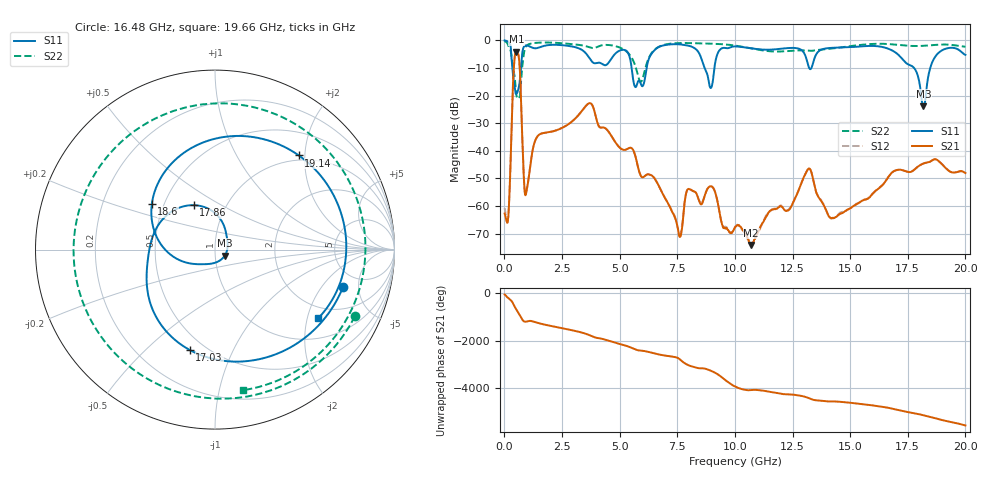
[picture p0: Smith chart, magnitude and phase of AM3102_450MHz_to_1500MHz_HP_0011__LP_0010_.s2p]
!Agilent Technologies,E8364B,MY43040894,A.07.50.67
!Agilent E8364B: A.07.50.67
!Date: Thursday, January 11, 2018 05:30:21
!Correction: S11(Full 2 Port(1,2))
!S21(Full 2 Port(1,2))
!S12(Full 2 Port(1,2))
!S22(Full 2 Port(1,2))
!S2P File: Measurements: S11, S21, S12, S22:
# Hz S  dB  R 50
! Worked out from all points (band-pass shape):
!   1601 points, 10 MHz to 20 GHz, reference 50 ohm
!   highest |S21| = -4.07 dB at 522.2 MHz (marker M1); lowest = -74.1 dB at 10.7 GHz (marker M2)
!   |S21| within 3 dB of the highest: 436.3 MHz to 640 MHz (203.6 MHz wide, 37.8 % of centre)
!   lowest |S11| = -23.9 dB at 18.18 GHz (marker M3), VSWR 1.14, Z = 55.7 - j3.69 ohm
!   |S11| at or under -10 dB: 5.521 GHz to 6.172 GHz (650.8 MHz wide, 11.1 % of centre); 8.685 GHz to 9.111 GHz (426.6 MHz wide, 4.79 % of centre); 17.77 GHz to 18.48 GHz (702.7 MHz wide, 3.88 % of centre)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
!   |S22| runs from -21.1 to -0.3 dB; largest |S21 - S12| = 0.0015
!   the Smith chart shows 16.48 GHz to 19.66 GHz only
!   S11 on the Smith chart (normalised r, x): 16.48 GHz: 3.58, -3.32; 17.03 GHz: 0.41, -0.69; 17.86 GHz: 0.70, +0.38; 18.6 GHz: 0.43, +0.27; 19.14 GHz: 0.91, +1.88; 19.66 GHz: 1.61, -2.35
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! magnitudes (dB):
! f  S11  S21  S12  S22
! 10 MHz  -0.1  -62.7  -60.8  -0.3
! 172.4 MHz  -0.6  -63.7  -63.7  -2.0
! 522.2 MHz  -18.7  -4.1  -4.1  -19.9
! 947 MHz  -1.9  -55.2  -55.3  -2.1
! 3.346 GHz  -3.4  -25.7  -25.7  -1.8
! 5.707 GHz  -16.9  -42.7  -42.7  -10.0
! 6.682 GHz  -2.5  -52.4  -52.4  -2.4
! 7.606 GHz  -1.5  -71.2  -70.4  -1.0
! 8.956 GHz  -17.3  -52.8  -52.8  -1.2
! 10.01 GHz  -2.2  -67.7  -67.6  -1.9
! 10.7 GHz  -2.9  -74.1  -74.5  -2.9
! 13.34 GHz  -9.6  -48.4  -48.4  -3.8
! 14.22 GHz  -2.7  -64.3  -64.5  -3.0
! 16.48 GHz  -2.6  -51.7  -51.7  -1.3
! 16.68 GHz  -3.1  -49.2  -49.3  -1.4
! 17.03 GHz  -4.8  -47.0  -47.0  -1.6
! 17.86 GHz  -11.2  -46.2  -46.2  -2.1
! 18.18 GHz  -23.9  -44.6  -44.6  -2.0
! 18.6 GHz  -7.2  -43.2  -43.3  -1.7
! 19.14 GHz  -3.1  -46.2  -46.1  -1.5
! 19.66 GHz  -3.2  -47.6  -47.7  -2.0
! 20 GHz  -5.3  -48.1  -47.9  -2.3
